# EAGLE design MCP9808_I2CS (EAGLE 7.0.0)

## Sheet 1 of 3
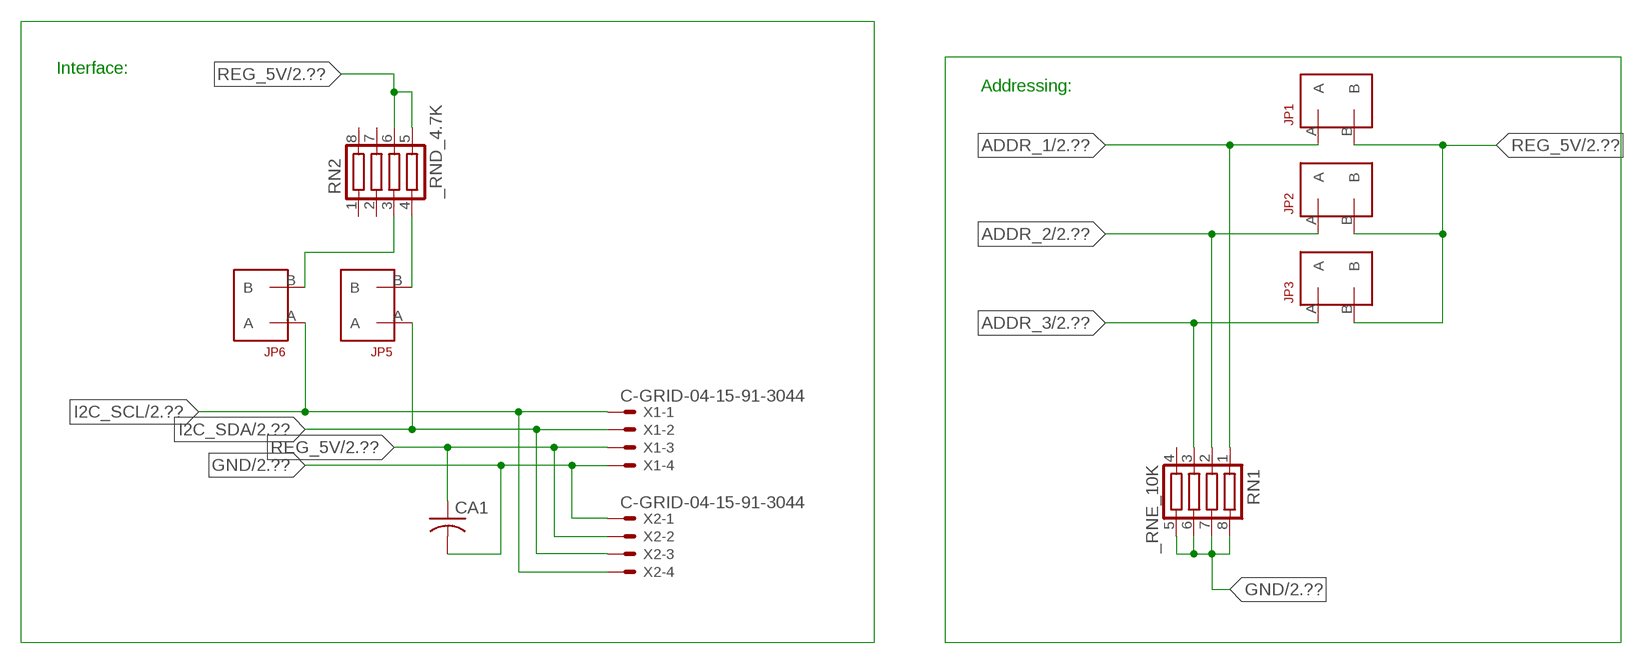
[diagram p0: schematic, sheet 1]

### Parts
CA1  CC1206KRX7R9BB104  [.1UF]
JP1  JUMPER_1X2_2MM  [JUMPER_1X2_2MM]
JP2  JUMPER_1X2_2MM  [JUMPER_1X2_2MM]
JP3  JUMPER_1X2_2MM  [JUMPER_1X2_2MM]
JP5  JUMPER_1X2_2MM  [JUMPER_1X2_2MM]
JP6  JUMPER_1X2_2MM  [JUMPER_1X2_2MM]
RN1  _RNE_10K  [RNE]
RN2  _RND_4.7K  [RND]
X1  C-GRID-04-15-91-3044  [15-91-04]
X2  C-GRID-04-15-91-3044  [15-91-04]

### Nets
ADDR_1: JP1.A RN1.1 ; also sheet 2
ADDR_2: JP2.A RN1.2 ; also sheet 2
ADDR_3: JP3.A RN1.3 ; also sheet 2
GND: CA1.2 RN1.5 RN1.6 RN1.7 RN1.8 X1.4 X2.1 ; also sheet 2,3
I2C_SCL: JP6.A X1.1 X2.4 ; also sheet 2
I2C_SDA: JP5.A X1.2 X2.3 ; also sheet 2
N$1: JP6.B RN2.3
N$2: JP5.B RN2.4
REG_5V: CA1.1 JP1.B JP2.B JP3.B RN2.5 RN2.6 X1.3 X2.2 ; also sheet 2,3
Unconnected: RN1.4 RN2.1 RN2.2 RN2.7 RN2.8

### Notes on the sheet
- Interface:
- Addressing:

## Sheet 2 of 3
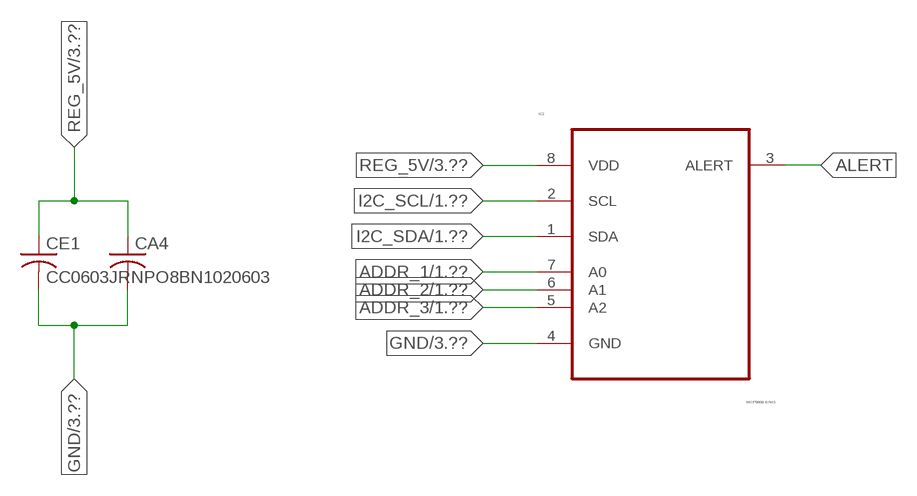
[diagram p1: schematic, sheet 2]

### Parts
CA4  CC1206KRX7R9BB104  [.1UF]
CE1  CC0603JRNPO8BN1020603  [CC0603JRNPO8BN102]
IC2  MCP9808-E/MS  [SOP65P490X110-8N]

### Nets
ADDR_1: IC2.7(A0) ; also sheet 1
ADDR_2: IC2.6(A1) ; also sheet 1
ADDR_3: IC2.5(A2) ; also sheet 1
ALERT: IC2.3(ALERT)
GND: CA4.2 CE1.2 IC2.4(GND) ; also sheet 1,3
I2C_SCL: IC2.2(SCL) ; also sheet 1
I2C_SDA: IC2.1(SDA) ; also sheet 1
REG_5V: CA4.1 CE1.1 IC2.8(VDD) ; also sheet 1,3

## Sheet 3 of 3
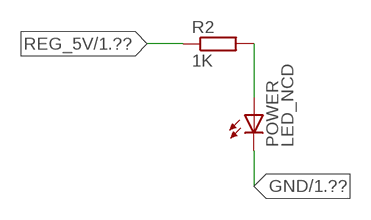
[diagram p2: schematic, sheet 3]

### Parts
POWER  LED_NCD  [CHIPLED_0603]
R2  1K  RESISTOR_SMT-0402  [R402]

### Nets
GND: POWER.C ; also sheet 1,2
N$3: POWER.A R2.2
REG_5V: R2.1 ; also sheet 1,2

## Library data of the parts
CA1 = NCD_ULTIMATE_LIBRARY:CC1206KRX7R9BB104: Capacitor CA .1uF 50V SMT C1206K CC1206KRX7R9BB104
CA4 = NCD_ULTIMATE_LIBRARY (2):CC1206KRX7R9BB104: Capacitor CA .1uF 50V SMT C1206K CC1206KRX7R9BB104
CE1 = NCD_ULTIMATE_LIBRARY (2):CC0603JRNPO8BN102: Capacitor CE 1uF SMT CC0603JRNPO8BN102 0603
IC2 = NCD_ULTIMATE_KAMNA:MCP9808-E/MS: Digital Temperature Sensor,MSOP-8; MPN: MCP9808-E/MS; OC_FARNELL: 2080523; OC_NEWARK: 89T8871; PACKAGE: MSOP-8; SUPPLIER: MICROCHIP
JP1-JP3 JP5 JP6 = NCD_ULTIMATE_CONNECTORS:JUMPER_1X2_2MM
POWER = NCD_ULTIMATE_LIBRARY:LED_NCD: LED Digikey 754-1132-2-ND/APT2012SRCPRV
R2 = NCD_ULTIMATE_LIBRARY:RESISTOR_SMT: NCD Resistor
RN1 = NCD_ULTIMATE_LIBRARY:_RNE_10K: Resistor Array RNE SMT 10K x 4 Single Resistor Source: http://www.ctscorp.com/components/Datasheets/CTSChipArrayDs.pdf Digikey 742C083103JPTR-ND/742C083103JP; OC_FARNELL: unknown; OC_NEWARK: unknown
RN2 = NCD_ULTIMATE_LIBRARY:_RND_4.7K: Resistor Array RND SMT 4.7K x 4 Single Resistor Source: http://www.ctscorp.com/components/Datasheets/CTSChipArrayDs.pdf Digikey 742C083472JPTR-ND/742C083472JP; OC_FARNELL: unknown; OC_NEWARK: unknown
X1 X2 = NCD_ULTIMATE_CONNECTORS:C-GRID-04: CONNECTOR 4-Pos I2C wire to board 2.54 mm (0.100") pitch header Digikey WM1342-ND/0015912045; OC_FARNELL: unknown; OC_NEWARK: unknown

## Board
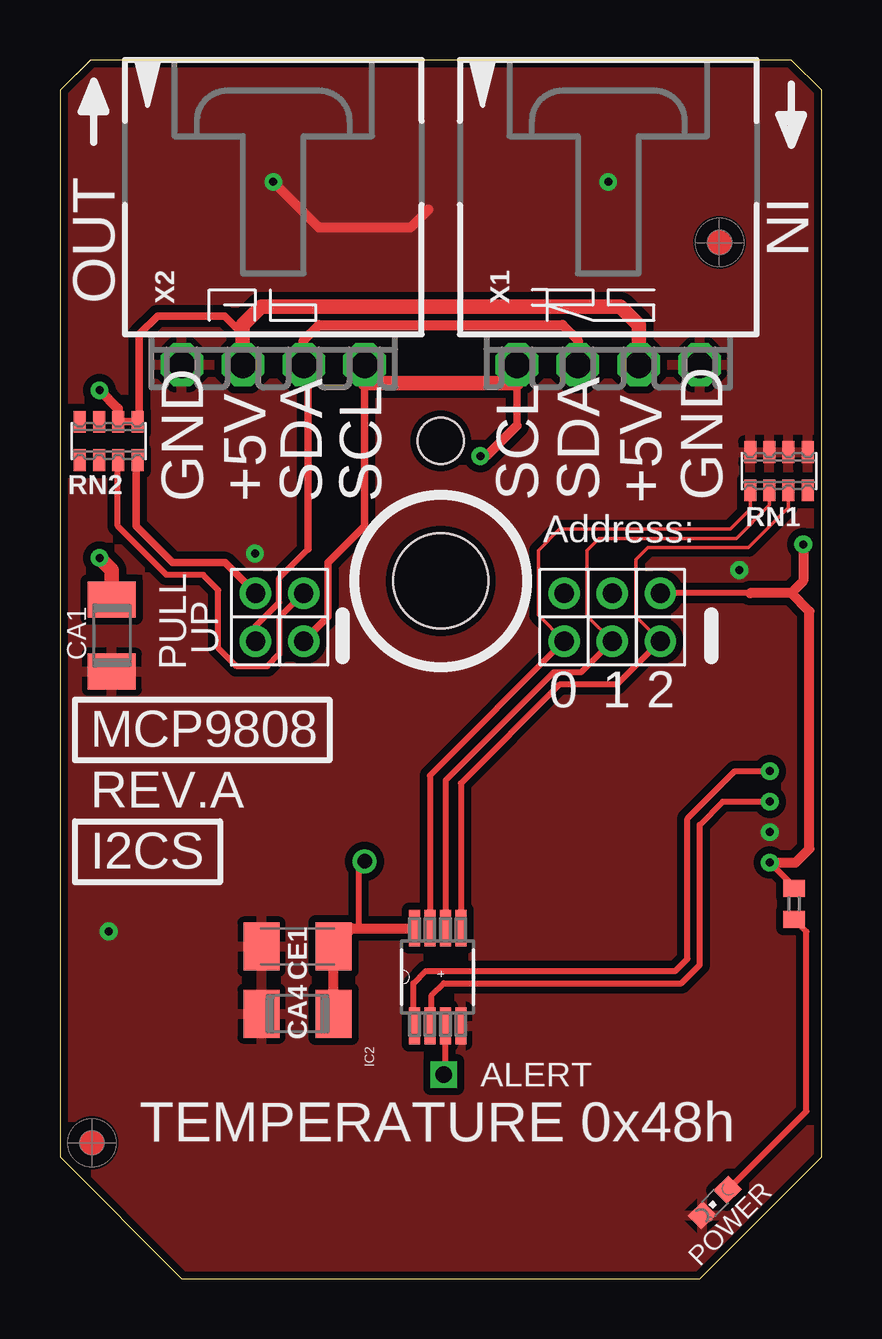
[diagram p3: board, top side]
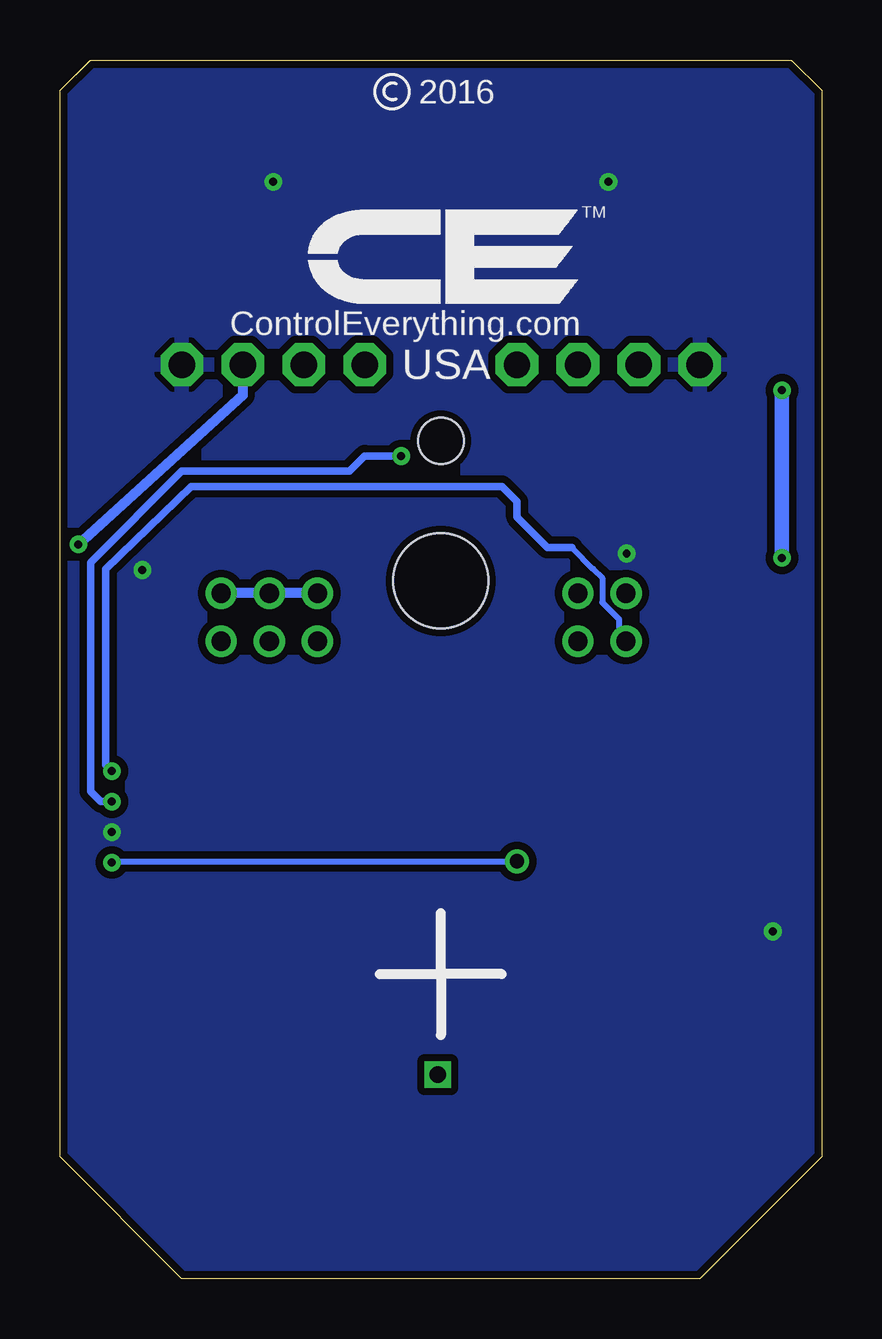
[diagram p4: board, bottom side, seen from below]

Size 31.75 x 50.8 mm. Coordinates in mm from the lower left corner, seen from the top.
Outline: 32 segments
Copper layers (1*16): Top 0.035mm / dielectric 1.5mm / Bottom 0.035mm
Design rules "default": minimum track width 5mil, minimum drill 24mil, track to track 5mil, track to pad 5mil, pad to pad 5mil, via to via 5mil, smd to smd 5mil, copper to edge 10mil, drill to drill 8mil, minimum pad ring 10mil, minimum via ring 8mil, stop-mask expansion 2mil, vias tented up to drill 0mil, thermal gap 10mil
Holes 3.96 mm at 15.88,29.08
Holes 1.91 mm at 15.88,34.92

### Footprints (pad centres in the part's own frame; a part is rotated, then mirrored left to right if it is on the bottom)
.1UF = smd 1.5 x 2: 1 -1.5,0; 2 1.5,0
CC0603JRNPO8BN102 = smd 1.5 x 2: 1 -1.5,0; 2 1.5,0
SOP65P490X110-8N = smd 1.524 x 0.457: 1 -2.032,0.965; 2 -2.032,0.33; 3 -2.032,-0.33; 4 -2.032,-0.965; 5 2.032,-0.965; 6 2.032,-0.33; 7 2.032,0.33; 8 2.032,0.965
JUMPER_1X2_2MM = drill 0.8: A 0,2; B 0,0
CHIPLED_0603 = smd 0.8 x 0.876: A 0,-0.75; C 0,0.75
R402 = smd 0.7 x 0.9: 1 -0.65,0; 2 0.65,0
RNE = smd 0.5 x 0.9: 1 -1.2,-0.8; 2 -0.4,-0.8; 3 0.4,-0.8; 4 1.2,-0.8; 5 1.2,0.8; 6 0.4,0.8; 7 -0.4,0.8; 8 -1.2,0.8
RND = smd 0.5 x 0.9: 1 -1.2,-0.8; 2 -0.4,-0.8; 3 0.4,-0.8; 4 1.2,-0.8; 5 1.2,0.8; 6 0.4,0.8; 7 -0.4,0.8; 8 -1.2,0.8
15-91-04 = drill 1.1 pad 1.778 octagon: 1 -3.81,-7.62; 2 -1.27,-7.62; 3 1.27,-7.62; 4 3.81,-7.62

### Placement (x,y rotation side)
CA1  2.16,26.81 270 top
CA4  9.91,11.05 180 top
CE1  9.91,13.84 180 top
IC2  15.75,12.57 90 top
JP1  21.02,28.58 180 top
JP2  23.03,28.58 180 top
JP3  25.03,28.58 180 top
JP5  8.15,28.58 180 top
JP6  10.16,28.58 180 top
POWER  27.3,3.18 135 top
R2  30.61,15.62 270 top
RN1  29.97,33.66 0 top
RN2  2.03,34.92 0 top
U$5  [VISION_REF10]  1.33,5.66 90 top
U$28  [VISION_REF10]  27.5,43.19 90 top
X1  22.86,45.72 0 top
X2  8.89,45.72 0 top

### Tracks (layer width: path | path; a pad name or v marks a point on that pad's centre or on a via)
ADDR_1
  Top 0.152: RN1.1 28.77,32.07 27.94,31.24 20.83,31.24 19.94,30.35 19.94,27.65 JP1.A
  Top 0.254: JP1.A 15.42,20.97 IC2.7
ADDR_2
  Top 0.152: RN1.2 29.57,32.24 28.19,30.86 22.48,30.86 21.97,30.35 21.97,27.63 JP2.A
  Top 0.254: JP2.A 21.72,25.27 20.57,25.27 16.08,20.78 IC2.6
ADDR_3
  Top 0.152: RN1.3 30.37,32.15 28.7,30.48 24.51,30.48 24,29.97 24,27.6 JP3.A
  Top 0.254: JP3.A 23.22,24.77 20.83,24.77 16.71,20.65 IC2.5
ALERT  (via drill 0.7)
  Top 0.254: v16,8.51 16.08,8.59 IC2.3
GND  (via drill 0.33)
  Top 0.406: 15.35,44.57 14.6,43.82 10.8,43.82 v8.89,45.72
  other vias: 22.86,45.72 29.59,18.62 2.03,14.48 8.13,30.23 28.32,29.54
  pour Top (isolate 0.305): -1.27,0 -1.27,50.8 33.02,50.8 33.02,0
  pour Bottom (isolate 0.305): -5.08,0 -5.08,50.8 35.56,50.8 35.56,0
I2C_SCL  (via drill 0.33)
  Top 0.254: IC2.2 15.49,10.62 15.49,11.81 16,12.32 25.91,12.32 26.67,13.08 26.67,18.92 27.63,19.89 v29.59,19.89
  Top 0.305: JP6.A 11.18,27.61 11.18,29.85 12.7,31.37 X2.4 | 19.05,35.56 X1.1
  Top 0.406: X2.4 12.7,37.34 | 19.05,37.34 X1.1 | 19.05,35.56 17.78,34.29 v17.53,34.29
  Top 0.61: 12.7,37.34 19.05,37.34
  Bottom 0.305: v29.59,19.89 30.05,19.89 30.48,20.32 30.48,29.85 26.67,33.66 19.69,33.66 19.05,34.29 v17.53,34.29
I2C_SDA  (via drill 0.33)
  Top 0.254: JP5.A 8.15,27.2 9.14,28.19 9.14,29.21 10.35,30.42 | IC2.1 14.73,10.59 14.73,12.32 15.24,12.83 25.65,12.83 26.16,13.34 26.16,19.18 28.14,21.16 v29.59,21.16
  Top 0.305: 10.35,30.42 10.35,37.91 X2.3
  Top 0.406: X2.3 10.16,39.12 10.8,39.75 20.96,39.75 21.59,39.12 X1.2
  Bottom 0.254: 10.41,30.48 9.52,29.59 9.14,29.21 9.14,28.19 8.45,27.5 8.45,26.87 JP5.A
  Bottom 0.305: 10.41,30.48 11.43,30.48 12.7,31.75 12.7,32.39 13.34,33.02 26.29,33.02 29.85,29.59 29.85,21.41 v29.59,21.16
N$1
  Top 0.254: JP6.B | JP6.B 9.14,27.56 9.14,26.04 8.64,25.53 7.37,25.53 6.6,26.29 6.6,28.7 5.97,29.34 4.45,29.34 2.41,31.37 2.41,34.11 RN2.3
N$2
  Top 0.305: JP5.B 6.88,29.85 4.7,29.85 3.18,31.37 3.18,34.07 RN2.4
N$3
  Top 0.254: POWER.A 31.12,6.99 31.12,14.46 R2.2
REG_5V  (via drill 0.33, 0.6)
  Top 0.254: v29.59,17.35 30.61,16.33 R2.1 | v12.7,17.4 12.45,17.15 12.45,14.61 | 28.77,28.58 | 28.77,28.58 JP3.B
  Top 0.305: 7.62,39.37 7.49,39.37 | RN2.6 RN2.5 3.3,35.8 3.3,39.37 4.06,40.13 6.86,40.13 7.62,39.37 | X2.2 7.62,39.37
  Top 0.406: v29.59,17.35 30.67,17.35 31.24,17.92 31.24,27.81 30.48,28.58 | v1.65,37.03 2.41,36.27 2.41,35.74 RN2.6 | 30.48,28.58 28.77,28.58 | v30.99,30.61 30.99,29.08 30.48,28.58 | X1.3 24.13,37.47 | CA4.1 CE1.1 12.17,14.61 12.45,14.61 IC2.8
  Top 0.61: X2.2 7.62,39.75 8.38,40.51 23.37,40.51 24.13,39.75 X1.3 | CA1.1 2.16,29.54 v1.65,30.05
  Bottom 0.254: v29.59,17.35 29.54,17.4 v12.7,17.4
  Bottom 0.406: 24.16,38.08 24.13,37.47 | 24.13,37.47 24.13,36.83 v30.99,30.61 | JP1.B JP2.B JP3.B | 24.13,37.47 X1.3
  Bottom 0.61: v1.65,30.05 v1.65,37.03

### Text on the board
tNames: IN | OUT | GND | +5V | SDA | SCL | SCL | SDA | +5V | GND | Address: | UP | PULL | 0 | 1 | 2 | MCP9808 | REV.A | I2CS | ALERT | TEMPERATURE 0x48h
bNames: 2016 | TM | ControlEverything.com | USA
